(* Logix 5000 DataType export; software revision 16.04 *)

TYPE Motion_Task :
STRUCT
   Accel : LINT;   // MT.ACC Acceleration
   ControlWord : DINT;   // MT.CNTL
   Decel : LINT;   // MT.DEC
   Delay : INT;   // MT.TNEXT Delay before executing next task
   NextNum : SINT;   // MT.TNEXT Number of next task to execute
   Position : LINT;   // MT.P Target Position
   Num : SINT;   // MT.NUM Number of this task in the table
   Velocity : LINT;   // MT.V Target Velocity
   Set : SINT;   // Used to command a set of the MT. Should always equal 1
END_STRUCT
END_TYPE
